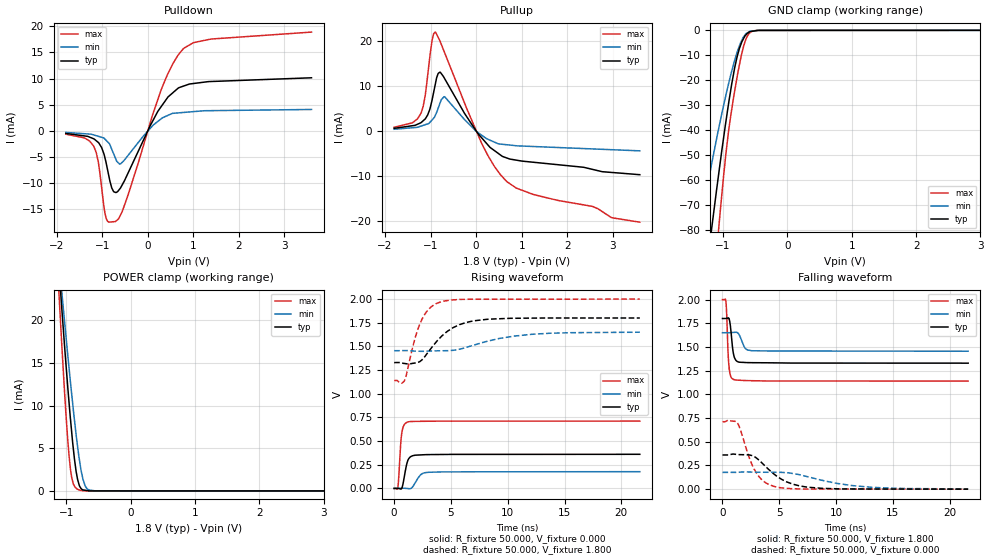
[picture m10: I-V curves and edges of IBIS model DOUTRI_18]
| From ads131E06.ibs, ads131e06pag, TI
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|   DOUTRI 1.8V Model
[Model]   DOUTRI_18
Model_type   I/O
|for ADS1291, ADS1292, ADS1294, ADS1296, and ADS1298 products
|Signals   DOUT, _DRDY
Vinl = .36
Vinh = 1.44
Vmeas = 0.9
Vref = 0.9
Cref = 2pF
Rref = 50
|   typ   min   max
|   (nom PVT)   (Fast PVT)   (slow PVT)
|C_comp from frequency sweep method (F=64MHz)
|   (Hight Z)
|C_comp   3.2922120e-12   2.4308820e-12   4.0512090e-12
|   (ON state)
|C_comp   6.1104920e-12   5.1552980e-12   6.0686990e-12
|   (OFF state)
|C_comp   5.4833710e-12   4.7517900e-12   6.1905060e-12
|C_comp from LC tank measurement(L=1nH)
|   (HIGH Z)
|C_comp   2.595E-12   1.959E-12   3.251E-12
|   (ON state)
C_comp   2.655E-12   2.042E-12   3.297E-12
|   (OFF state)
|C_comp   2.704E-12   2.129E-12   3.327E-12
| Where   nom PVT is  Nominal Process, 1.8V, 27C
|   Fast PVT is Strong Process, 2V, -40C
|   Slow PVT is Weak Process, 1.65V, 85C
[Voltage Range]   1.8   1.65   2
[Temperature Range]   27   85   -40
[Pullup Reference]   1.8   1.65   2
[Pulldown Reference]   0   0   0
[Power Clamp Reference]   1.8   1.65   2
[GND Clamp Reference]   0   0   0
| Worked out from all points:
|   slope of the pulldown table from 0 to 0.27 V, typ, clamps not added: 62.2 ohm
|   slope of the pullup table from 0 to 0.27 V, typ, clamps not added: 82.6 ohm
|   GND clamp passes 1 mA (typ) near -0.61 V on its own axis
|   POWER clamp passes 1 mA (typ) near -0.81 V on its own axis
|   falling waveform, R_fixture 50.000, V_fixture 1.800: 20-80 % time 265ps typ, 413ps min, 183ps max; typ from 1.8 V to 1.33 V
|   rising waveform, R_fixture 50.000, V_fixture 0.000: 20-80 % time 366ps typ, 580ps min, 238ps max; typ from 0 V to 0.361 V
|   rising waveform, R_fixture 50.000, V_fixture 1.800: 20-80 % time 2.43ns typ, 4.26ns min, 1.35ns max; typ from 1.33 V to 1.8 V
|   falling waveform, R_fixture 50.000, V_fixture 0.000: 20-80 % time 2.39ns typ, 4.37ns min, 1.42ns max; typ from 0.361 V to 0 V
[Pulldown]
|   Voltage   I(typ)   I(min)   I(max)
-1.8V     -493.2uA   -302.1uA   -631.4uA
-1.191V   -1.507mA   -773.1uA   -2.888mA
-1.088V   -2.206mA   -1.037mA   -5.859mA
-918.3mV  -5.959mA   -1.782mA   -16.59mA
-791.8mV  -10.89mA   -3.506mA   -17.41mA
-713.5mV  -11.75mA   -5.158mA   -17.34mA
-595.9mV  -10.87mA   -6.296mA   -16.04mA
311.8mV   4.852mA    2.432mA    8.246mA
556.6mV   7.33mA     3.353mA    12.93mA
781.6mV   8.551mA    3.515mA    15.71mA
1.387V    9.431mA    3.861mA    17.55mA
3.595V    10.14mA    4.088mA    18.88mA
[GND Clamp]
|   Voltage   I(typ)   I(min)   I(max)
-1.8V     -217.9mA   -147.2mA   -309mA
-1.352V   -116.5mA   -77.88mA   -165.9mA
-1.176V   -79.18mA   -53.33mA   -111.4mA
-1.072V   -58.33mA   -39.81mA   -80.57mA
-1.047V   -53.6mA    -36.84mA   -73.57mA
-954.1mV  -36.31mA   -25.8mA    -49.12mA
-884.3mV  -24.54mA   -18.23mA   -34.87mA
-777.9mV  -10.26mA   -8.507mA   -18.18mA
-720.8mV  -5.523mA   -4.648mA   -10.62mA
-640.4mV  -1.698mA   -1.238mA   -3.306mA
-457.1mV  -23.74uA   -48.96uA   -23.16uA
3.595V    0A         0A         0A
[Pullup]
|   Voltage   I(typ)   I(min)   I(max)
-1.8V     604.7uA    404.2uA    846.7uA
-1.402V   1.187mA    737.9uA    1.825mA
-1.212V   1.853mA    1.104mA    3.943mA
-1.121V   2.672mA    1.413mA    7.738mA
-1.019V   4.767mA    1.898mA    16.29mA
-964mV    7.081mA    2.525mA    20.39mA
-898.9mV  10.31mA    3.436mA    22.08mA
-797.4mV  13.14mA    6.105mA    20.16mA
-689.1mV  11.65mA    7.637mA    17.42mA
133mV     -1.636mA   -1mA       -2.971mA
666.3mV   -5.981mA   -3.046mA   -11.19mA
3.595V    -9.731mA   -4.412mA   -20.33mA
[POWER Clamp]
|   Voltage   I(typ)   I(min)   I(max)
-1.8V     105.8mA    89.96mA    127.6mA
-1.113V   25.83mA    26.79mA    22.81mA
-1.074V   21.62mA    23.5mA     17.42mA
-1.063V   20.53mA    22.65mA    16.04mA
-1.008V   15.01mA    18.26mA    9.176mA
-959mV    10.37mA    14.42mA    4.162mA
-935.7mV  8.339mA    12.65mA    2.489mA
-895.8mV  5.179mA    9.757mA    897.6uA
-829.8mV  1.498mA    5.427mA    205.4uA
-743.9mV  121.6uA    1.401mA    35.91uA
-649.9mV  11.07uA    108.9uA    6.676uA
3.595V    0A         0A         0A
[Ramp]
R_load = 50
|   typ   min   max
dV/dt_r   0.216435/3.62674e-010   0.10679/5.69775e-010  0.426814/2.37203e-010
dV/dt_f   0.282365/2.61418e-010  0.116757/4.07543e-010  0.515701/1.82597e-010
[Falling Waveform]
R_fixture = 50.000
V_fixture = 1.800
V_fixture_min = 1.650
V_fixture_max = 2.000
C_fixture = 0.000
|  time   V(typ)   V(min)   V(max)
0s        1.8V       1.65V      2V
294.8ps   1.8V       1.65V      1.986V
370.2ps   1.802V     1.65V      1.845V
495.5ps   1.806V     1.65V      1.431V
585.2ps   1.795V     1.65V      1.279V
1.001ns   1.409V     1.653V     1.155V
1.305ns   1.346V     1.652V     1.15V
2ns       1.336V     1.486V     1.145V
2.579ns   1.334V     1.46V      1.144V
21.63ns   1.329V     1.455V     1.14V
[Rising Waveform]
R_fixture = 50.000
V_fixture = 0.000
V_fixture_min = 0.000
V_fixture_max = 0.000
C_fixture = 0.000
|  time   V(typ)   V(min)   V(max)
0s        3.353uV    2.262mV    -784.3nV
331.4ps   195.9uV    2.301mV    13.35mV
408.5ps   -425.7uV   2.31mV     125.2mV
591.4ps   -6.333mV   2.332mV    492.5mV
716ps     17.29mV    2.347mV    614.2mV
1.197ns   293.5mV    -894.9uV   702.5mV
1.535ns   340.7mV    4.715mV    707mV
2.361ns   354.5mV    147.3mV    709.1mV
3.049ns   357.6mV    170.8mV    710mV
21.63ns   360.7mV    177.2mV    711.4mV
[Rising Waveform]
R_fixture = 50.000
V_fixture = 1.800
V_fixture_min = 1.650
V_fixture_max = 2.000
C_fixture = 0.000
|  time   V(typ)   V(min)   V(max)
0s        1.329V     1.455V     1.14V
898.8ps   1.32V      1.456V     1.136V
1.819ns   1.324V     1.45V      1.577V
2.354ns   1.349V     1.448V     1.762V
3.059ns   1.449V     1.451V     1.895V
4.006ns   1.586V     1.454V     1.966V
5.732ns   1.729V     1.47V      1.996V
8.013ns   1.784V     1.549V     1.998V
12.41ns   1.799V     1.631V     1.999V
21.63ns   1.8V       1.65V      2V
[Falling Waveform]
R_fixture = 50.000
V_fixture = 0.000
V_fixture_min = 0.000
V_fixture_max = 0.000
C_fixture = 0.000
|  time   V(typ)   V(min)   V(max)
0s        360.7mV    177.2mV    711.4mV
1.3ns     365.7mV    178mV      700.4mV
2.411ns   359.5mV    180.9mV    315.1mV
2.901ns   336.3mV    178.8mV    187.6mV
3.626ns   259mV      178.4mV    82.78mV
4.547ns   158.2mV    177.9mV    28.58mV
6.243ns   51.12mV    163.9mV    4.221mV
8.768ns   8.5mV      93.44mV    1.399mV
13.27ns   1.832mV    19.14mV    909.4uV
21.63ns   3.353uV    2.262mV    -784.3nV
